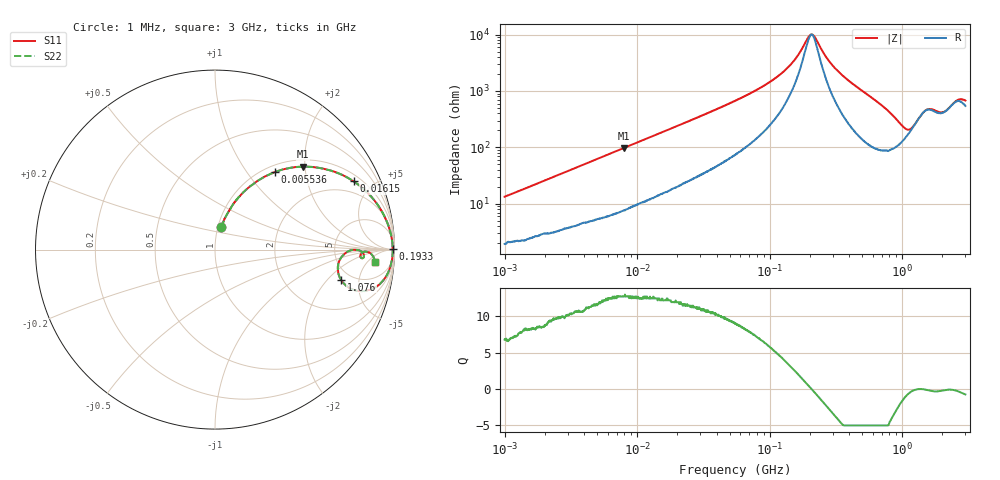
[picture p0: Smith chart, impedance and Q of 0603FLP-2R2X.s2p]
!s-Parameter Generated by FASTRON Sdn. Bhd.
!FASTRON P/N : 0603FLP-2R2X
!Keysight Technologies: E4991B_MY54100416_A.01.15
!Date: Tue Dec 02 13:02:51 2025
!Version  :Rev00  Tue Dec 02 13:02:51 2025
!Data & Calibration Information:
!Freq  S11  S21  S12  S22
!PortZ  Port1:50+j0  Port2:50+j0
!When reading reference impedance value at option line is always used.
! Remarks : This data is being provided solely for informational purposes.
# Hz S dB R 50
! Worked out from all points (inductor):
!   1601 points, 1 MHz to 3 GHz, reference 50 ohm
!   read as one part in series: L = 2.08 uH near 1.041 MHz
!   highest Q = 12.7 at 7.978 MHz (marker M1), where L = 1.95 uH
!   self-resonance near 207.2 MHz
!   S11 on the Smith chart (normalised r, x): 1 MHz: 1.04, +0.27; 5.536 MHz: 1.11, +1.38; 16.15 MHz: 1.32, +3.87; 193.3 MHz: open; 1.076 GHz: 4.10, -2.86; 3 GHz: 12, -8
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1000000  -17.70 74.2  -0.24 -7.4  -0.24 -7.4  -17.70 74.2
2215843  -11.50 68.5  -0.58 -15.4  -0.58 -15.4  -11.50 68.5
3804036  -7.57 60.0  -1.21 -24.6  -1.21 -24.6  -7.57 60.0
5536492  -5.24 52.2  -2.01 -33.0  -2.01 -33.0  -5.24 52.2
7977711  -3.42 43.2  -3.26 -42.3  -3.26 -42.3  -3.42 43.2
1.447069e7  -1.52 28.6  -6.37 -56.8  -6.37 -56.8  -1.52 28.6
1.615473e7  -1.30 26.2  -7.07 -59.1  -7.07 -59.1  -1.30 26.2
5.504702e7  -0.23 8.3  -16.80 -75.4  -16.80 -75.4  -0.23 8.3
1.232024e8  -0.10 2.7  -26.40 -74.3  -26.40 -74.3  -0.10 2.7
1.582265e8  -0.09 1.4  -31.80 -65.3  -31.80 -65.3  -0.09 1.4
1.93289e8  -0.09 0.3  -38.70 -31.3  -38.70 -31.3  -0.09 0.3
2.083556e8  -0.09 -0.0  -40.10 2.8  -40.10 2.8  -0.09 -0.0
2.75743e8  -0.09 -1.5  -31.20 67.4  -31.20 67.4  -0.09 -1.5
3.436571e8  -0.10 -2.8  -26.20 75.0  -26.20 75.0  -0.10 -2.8
7.925923e8  -0.60 -12.2  -13.30 66.1  -13.30 66.1  -0.60 -12.2
9.538021e8  -1.58 -16.1  -10.30 49.3  -10.30 49.3  -1.58 -16.1
1.075512e9  -2.84 -13.4  -9.31 29.2  -9.31 29.2  -2.84 -13.4
1.340405e9  -2.29 -0.1  -12.70 0.4  -12.70 0.4  -2.29 -0.1
1.542004e9  -1.67 -1.4  -15.10 6.7  -15.10 6.7  -1.67 -1.4
2.020405e9  -1.83 -2.3  -14.30 9.6  -14.30 9.6  -1.83 -2.3
2.607784e9  -1.15 -2.0  -17.90 13.7  -17.90 13.7  -1.15 -2.0
3e9  -1.00 -4.5  -17.60 32.1  -17.60 32.1  -1.00 -4.5
